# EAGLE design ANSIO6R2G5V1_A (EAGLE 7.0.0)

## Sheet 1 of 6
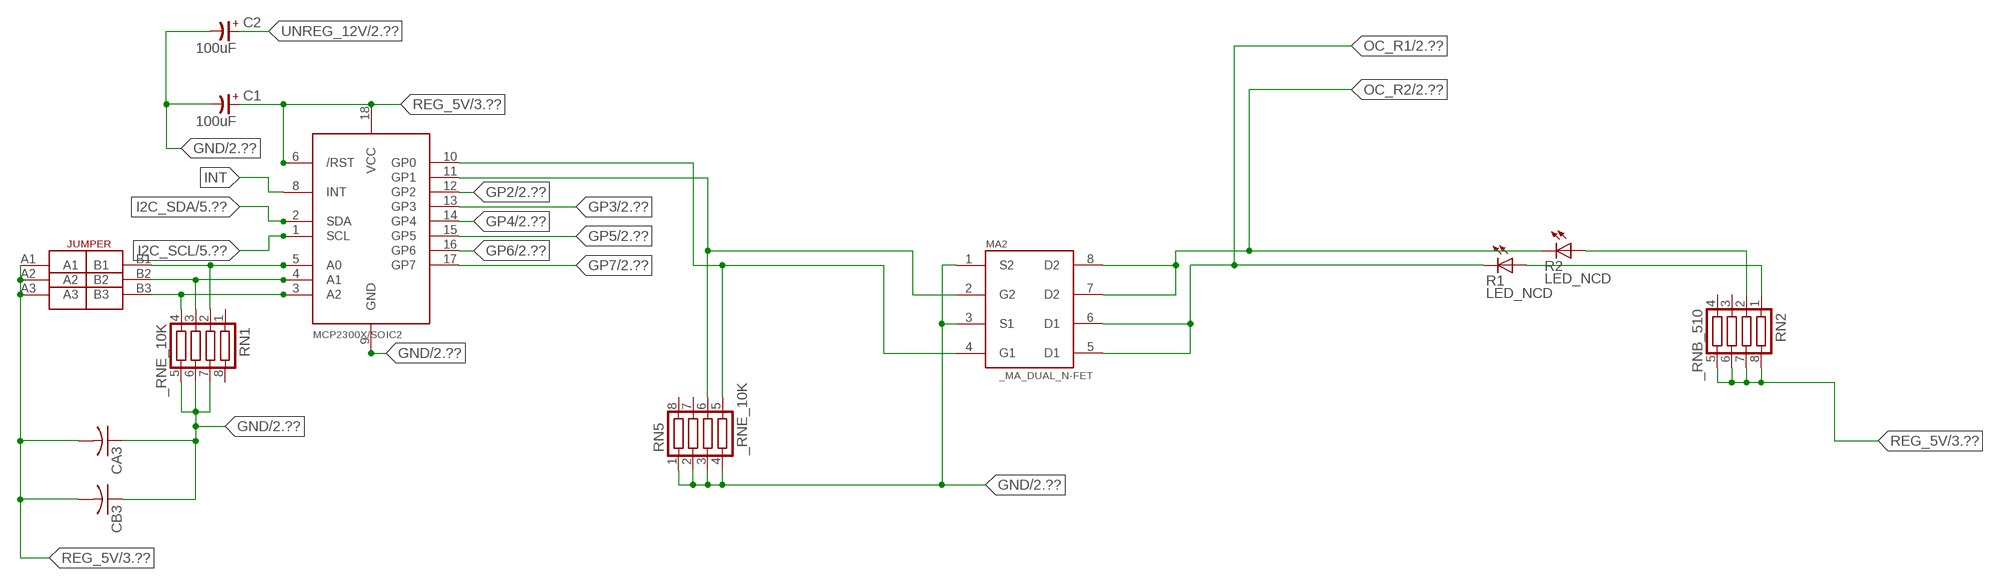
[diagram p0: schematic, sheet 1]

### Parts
C1  100uF  CP-E-025X060  [E-025X060]
C2  100uF  CP-E-025X060  [E-025X060]
CA3  CC1206KRX7R9BB104C1206K  [CC1206KRX7R9BB104]
CB3  TMK316F106ZL-TC1206K  [TMK316F106ZL-T]
IC2  MCP2300X/SO  [SO18W]
MA2  _MA_DUAL_N-FET  [_MA_DUAL_N-FET]
R1  LED_NCD  [CHIPLED_0603]
R2  LED_NCD  [CHIPLED_0603]
RN1  _RNE_10K  [RNE]
RN2  _RNB_510  [RNB]
RN5  _RNE_10K  [RNE]
U$18  JUMPER_3X2  [JUMPER_3X2]

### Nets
GND: C1.- C2.- CA3.1 CB3.1 IC2.9(GND) MA2.1(S2) MA2.3(S1) RN1.5 RN1.6 RN1.7 RN5.1 RN5.2 RN5.3 RN5.4 ; also sheet 2,3,4,5,6
GP2: IC2.12(GP2) ; also sheet 2
GP3: IC2.13(GP3) ; also sheet 2
GP4: IC2.14(GP4) ; also sheet 2
GP5: IC2.15(GP5) ; also sheet 2
GP6: IC2.16(GP6) ; also sheet 2
GP7: IC2.17(GP7) ; also sheet 2
I2C_SCL: IC2.1(SCL) ; also sheet 5,6
I2C_SDA: IC2.2(SDA) ; also sheet 5,6
INT: IC2.8(INT)
N$6: IC2.5(A0) RN1.2 U$18.B1
N$7: IC2.4(A1) RN1.3 U$18.B2
N$8: IC2.3(A2) RN1.4 U$18.B3
N$22: IC2.11(GP1) MA2.2(G2) RN5.6
N$23: IC2.10(GP0) MA2.4(G1) RN5.5
N$31: R2.A RN2.2
N$32: R1.A RN2.1
OC_R1: MA2.5(D1) MA2.6(D1) R1.C ; also sheet 2
OC_R2: MA2.7(D2) MA2.8(D2) R2.C ; also sheet 2
REG_5V: C1.+ CA3.2 CB3.2 IC2.6(/RST) IC2.18(VCC) RN2.5 RN2.6 RN2.7 RN2.8 U$18.A1 U$18.A2 U$18.A3 ; also sheet 3,4,5,6
UNREG_12V: C2.+ ; also sheet 2,3
Unconnected: RN1.1 RN1.8 RN2.3 RN2.4 RN5.7 RN5.8

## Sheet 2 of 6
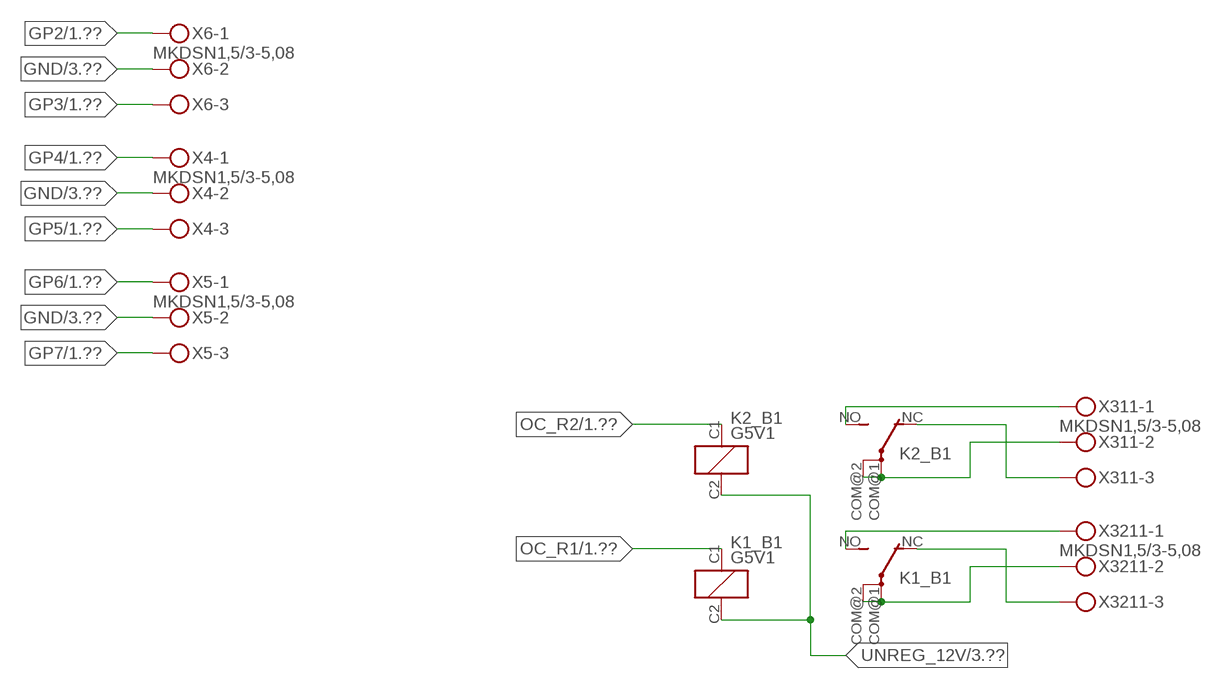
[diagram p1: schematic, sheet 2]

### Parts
K1_B1  G5V1  [G5V1]
K2_B1  G5V1  [G5V1]
X4  MKDSN1,5/3-5,08  [MKDSN1,5/3-5,08]
X5  MKDSN1,5/3-5,08  [MKDSN1,5/3-5,08]
X6  MKDSN1,5/3-5,08  [MKDSN1,5/3-5,08]
X311  MKDSN1,5/3-5,08  [MKDSN1,5/3-5,08]
X3211  MKDSN1,5/3-5,08  [MKDSN1,5/3-5,08]

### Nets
GND: X4.2 X5.2 X6.2 ; also sheet 1,3,4,5,6
GP2: X6.1 ; also sheet 1
GP3: X6.3 ; also sheet 1
GP4: X4.1 ; also sheet 1
GP5: X4.3 ; also sheet 1
GP6: X5.1 ; also sheet 1
GP7: X5.3 ; also sheet 1
N$221: K2_B1.NO(2:S) X311.1
N$222: K2_B1.NC(2:O) X311.3
N$223: K2_B1.COM@1(2:P) K2_B1.COM@2(2:P) X311.2
N$224: K1_B1.NO(2:S) X3211.1
N$225: K1_B1.NC(2:O) X3211.3
N$226: K1_B1.COM@1(2:P) K1_B1.COM@2(2:P) X3211.2
OC_R1: K1_B1.C1(1:C1) ; also sheet 1
OC_R2: K2_B1.C1(1:C1) ; also sheet 1
UNREG_12V: K1_B1.C2(1:C2) K2_B1.C2(1:C2) ; also sheet 1,3

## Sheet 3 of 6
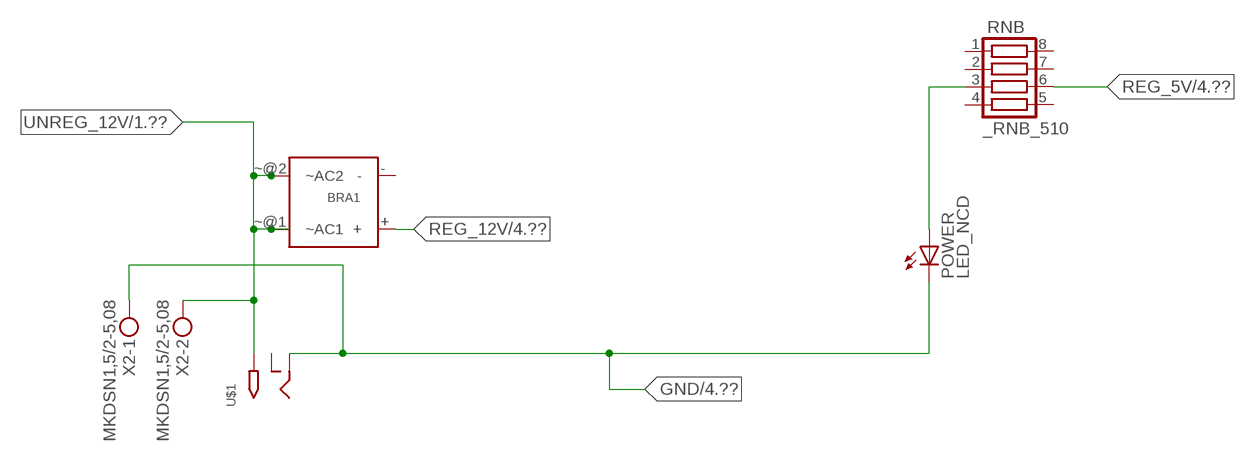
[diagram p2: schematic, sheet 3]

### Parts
BRA1  MB2S_  [MB2S]
POWER  LED_NCD  [CHIPLED_0603]
RNB  _RNB_510  [RNB]
U$1  2.1MMJACK  [PJ-102A]
X2  MKDSN1,5/2-5,08  [MKDSN1,5/2-5,08]

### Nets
GND: POWER.C U$1.RING X2.1 ; also sheet 1,2,4,5,6
N$2: POWER.A RNB.3
REG_5V: RNB.6 ; also sheet 1,4,5,6
REG_12V: BRA1.+ ; also sheet 4
UNREG_12V: BRA1.~@1(~AC1) BRA1.~@2(~AC2) U$1.TIP X2.2 ; also sheet 1,2
Unconnected: BRA1.- RNB.1 RNB.2 RNB.4 RNB.5 RNB.7 RNB.8 U$1.RING_SW

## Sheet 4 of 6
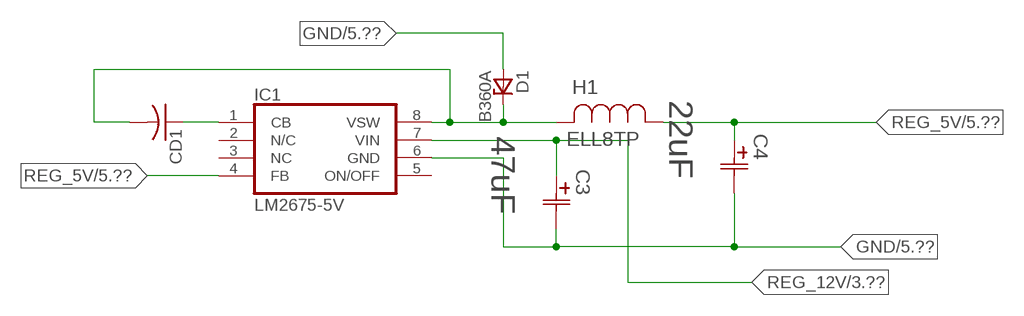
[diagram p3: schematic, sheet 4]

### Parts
C3  47uF  490-5463-6-NDCAP  [C2917(7343)-Y]
C4  22uF  490-5463-6-NDCAP  [C2917(7343)-Y]
CD1  _CD_10NF_50VC1206K  [_CD_10NF_50V]
D1  B360A  [DO214AC_ZENER]
H1  ELL8TP  [IND_ELL8TP]
IC1  LM2675-5V  LM2675  [SO-8]

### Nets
GND: C3.2(C2) C4.2(C2) D1.A IC1.6(GND) ; also sheet 1,2,3,5,6
N$1: CD1.2 D1.C H1.2 IC1.8(VSW)
N$3: CD1.1 IC1.1(CB)
REG_5V: C4.1(C1) H1.1 IC1.4(FB) ; also sheet 1,3,5,6
REG_12V: C3.1(C1) IC1.7(VIN) ; also sheet 3
Unconnected: IC1.2(N/C) IC1.5(ON/OFF)

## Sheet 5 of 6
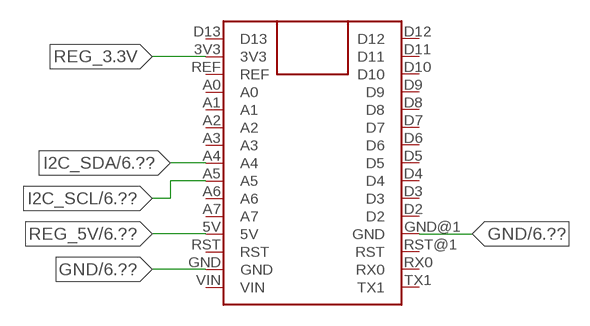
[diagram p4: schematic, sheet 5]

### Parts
FOR_NANO  ARDUINO_NANO  [ARDUINO_NANO]

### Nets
GND: FOR_NANO.GND FOR_NANO.GND@1(GND) ; also sheet 1,2,3,4,6
I2C_SCL: FOR_NANO.A5 ; also sheet 1,6
I2C_SDA: FOR_NANO.A4 ; also sheet 1,6
REG_3.3V: FOR_NANO.3V3
REG_5V: FOR_NANO.5V ; also sheet 1,3,4,6
Unconnected: FOR_NANO.A0 FOR_NANO.A1 FOR_NANO.A2 FOR_NANO.A3 FOR_NANO.A6 FOR_NANO.A7 FOR_NANO.D2 FOR_NANO.D3 FOR_NANO.D4 FOR_NANO.D5 FOR_NANO.D6 FOR_NANO.D7 FOR_NANO.D8 FOR_NANO.D9 FOR_NANO.D10 FOR_NANO.D11 FOR_NANO.D12 FOR_NANO.D13 FOR_NANO.REF FOR_NANO.RST FOR_NANO.RST@1(RST) FOR_NANO.RX0 FOR_NANO.TX1 FOR_NANO.VIN

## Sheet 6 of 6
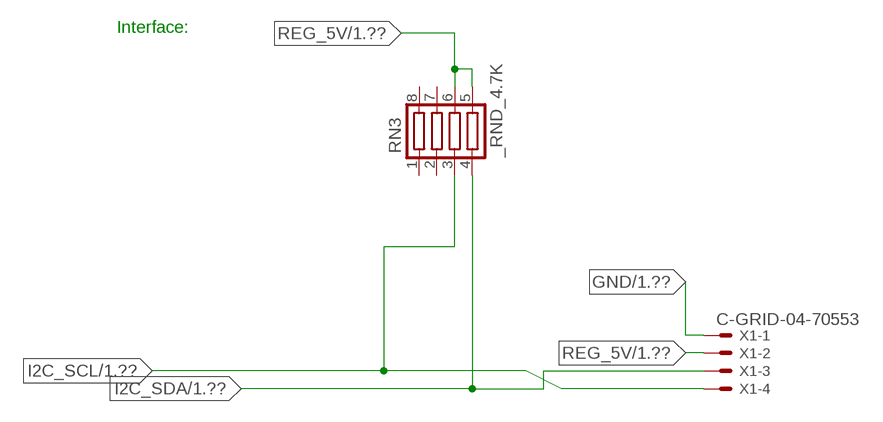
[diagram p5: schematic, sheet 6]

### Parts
RN3  _RND_4.7K  [RND]
X1  C-GRID-04-70553  [70553-04]

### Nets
GND: X1.1 ; also sheet 1,2,3,4,5
I2C_SCL: RN3.3 X1.4 ; also sheet 1,5
I2C_SDA: RN3.4 X1.3 ; also sheet 1,5
REG_5V: RN3.5 RN3.6 X1.2 ; also sheet 1,3,4,5
Unconnected: RN3.1 RN3.2 RN3.7 RN3.8

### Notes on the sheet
- Interface:

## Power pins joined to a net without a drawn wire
NC: IC1.3(NC)

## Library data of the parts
BRA1 = NCD_ULTIMATE_LIBRARY:MB2S: Bridge Rectifier BRA MB2S 200V 500ma Digikey MB2S-TPMSTR-ND/MB2S-TP
C1 C2 = NCD_ULTIMATE_LIBRARY:CP-: Capacitors All Kinds POLARIZED CAP
C3 C4 = NCD_ULTIMATE_bhaskar:490-5463-6-ND: NCD CAP
CA3 = NCD_ULTIMATE_LIBRARY:CC1206KRX7R9BB104: Capacitor CA .1uF 50V SMT C1206K CC1206KRX7R9BB104
CB3 = NCD_ULTIMATE_LIBRARY:TMK316F106ZL-T: Capacitor CB 10uF SMT 1206 TMK316F106ZL-T
CD1 = NCD_ULTIMATE_LIBRARY:_CD_10NF_50V: Capacitor 10nF SMT
D1 = NCD_ULTIMATE_bhaskar:B360A: NCD DIODE B350A/B360A
FOR_NANO = NCD_ULTIMATE_CONNECTORS:ARDUINO_NANO
H1 = NCD_ULTIMATE_bhaskar:ELL8TP: NCD coil
IC1 = NCD_ULTIMATE_bhaskar:LM2675: LM2675 NCD http://www.ti.com/lit/ds/symlink/lm2675.pdf
IC2 = NCD_ULTIMATE_LIBRARY:MCP2300X: Semiconductor Port Expander I/O 8-Bit I2C MCP23008 Inexpensive i2c i/o expander - 8 general purpose i/o pins with optional pullups
K1_B1 K2_B1 = NCD_ULTIMATE_LIBRARY:G5V1: RELAY 1 x switch, 0.5 A/125 V AC, 1 A/24 V DC , Omron
MA2 = NCD_ULTIMATE_LIBRARY:_MA_DUAL_N-FET: FET Dual N-Channel 8-SOIC NMOSFET Digikey 785-1064-2-ND/AO4842
POWER = NCD_ULTIMATE_bhaskar:LED_NCD
R1 R2 = NCD_ULTIMATE_LIBRARY:LED_NCD: LED Digikey 754-1132-2-ND/APT2012SRCPRV
RN1 RN5 = NCD_ULTIMATE_LIBRARY:_RNE_10K: Resistor Array RNE SMT 10K x 4 Single Resistor Source: http://www.ctscorp.com/components/Datasheets/CTSChipArrayDs.pdf Digikey 742C083103JPTR-ND/742C083103JP; OC_FARNELL: unknown; OC_NEWARK: unknown
RN2 RNB = NCD_ULTIMATE_LIBRARY:_RNB_510: Resistor Array RNB SMT 510 x 4 Single Resistor Source: http://www.ctscorp.com/components/Datasheets/CTSChipArrayDs.pdf Digikey 742C083511JPTR-ND/ 742C083511JP; OC_FARNELL: unknown; OC_NEWARK: unknown
RN3 = NCD_ULTIMATE_LIBRARY:_RND_4.7K: Resistor Array RND SMT 4.7K x 4 Single Resistor Source: http://www.ctscorp.com/components/Datasheets/CTSChipArrayDs.pdf Digikey 742C083472JPTR-ND/742C083472JP; OC_FARNELL: unknown; OC_NEWARK: unknown
U$1 = NCD_ULTIMATE_CONNECTORS:2.1MMJACK: 2.1mm x 5.5mm DC jack with internal switch. Digikey part #PJ-102A, 4UCON part #05537 By microbuilder.eu
U$18 = NCD_ULTIMATE_CONNECTORS:JUMPER_3X2
X1 = NCD_ULTIMATE_CONNECTORS:C-GRID-04: CONNECTOR 4-Pos I2C wire to board 2.54 mm (0.100") pitch header Digikey WM1342-ND/0015912045; OC_FARNELL: unknown; OC_NEWARK: unknown
X2 = NCD_ULTIMATE_CONNECTORS:MKDSN1,5/2-5,08: MKDSN 1,5/ 2-5,08 Printklemme
X4-X6 X311 X3211 = NCD_ULTIMATE_CONNECTORS:MKDSN1,5/3-5,08: MKDSN 1,5/ 3-5,08 Printklemme Nennstrom: 13,5 A Nennspannung: 250 V Rastermaß: 5,08 mm Polzahl: 3 Anschlussart: Schraubanschluss Montage: Löten Anschlussrichtung Leiter/Platine: 0 ° Artikelnummer: 1729131 Source: http://eshop.phoenixcontact.com .. 1729131.pdf

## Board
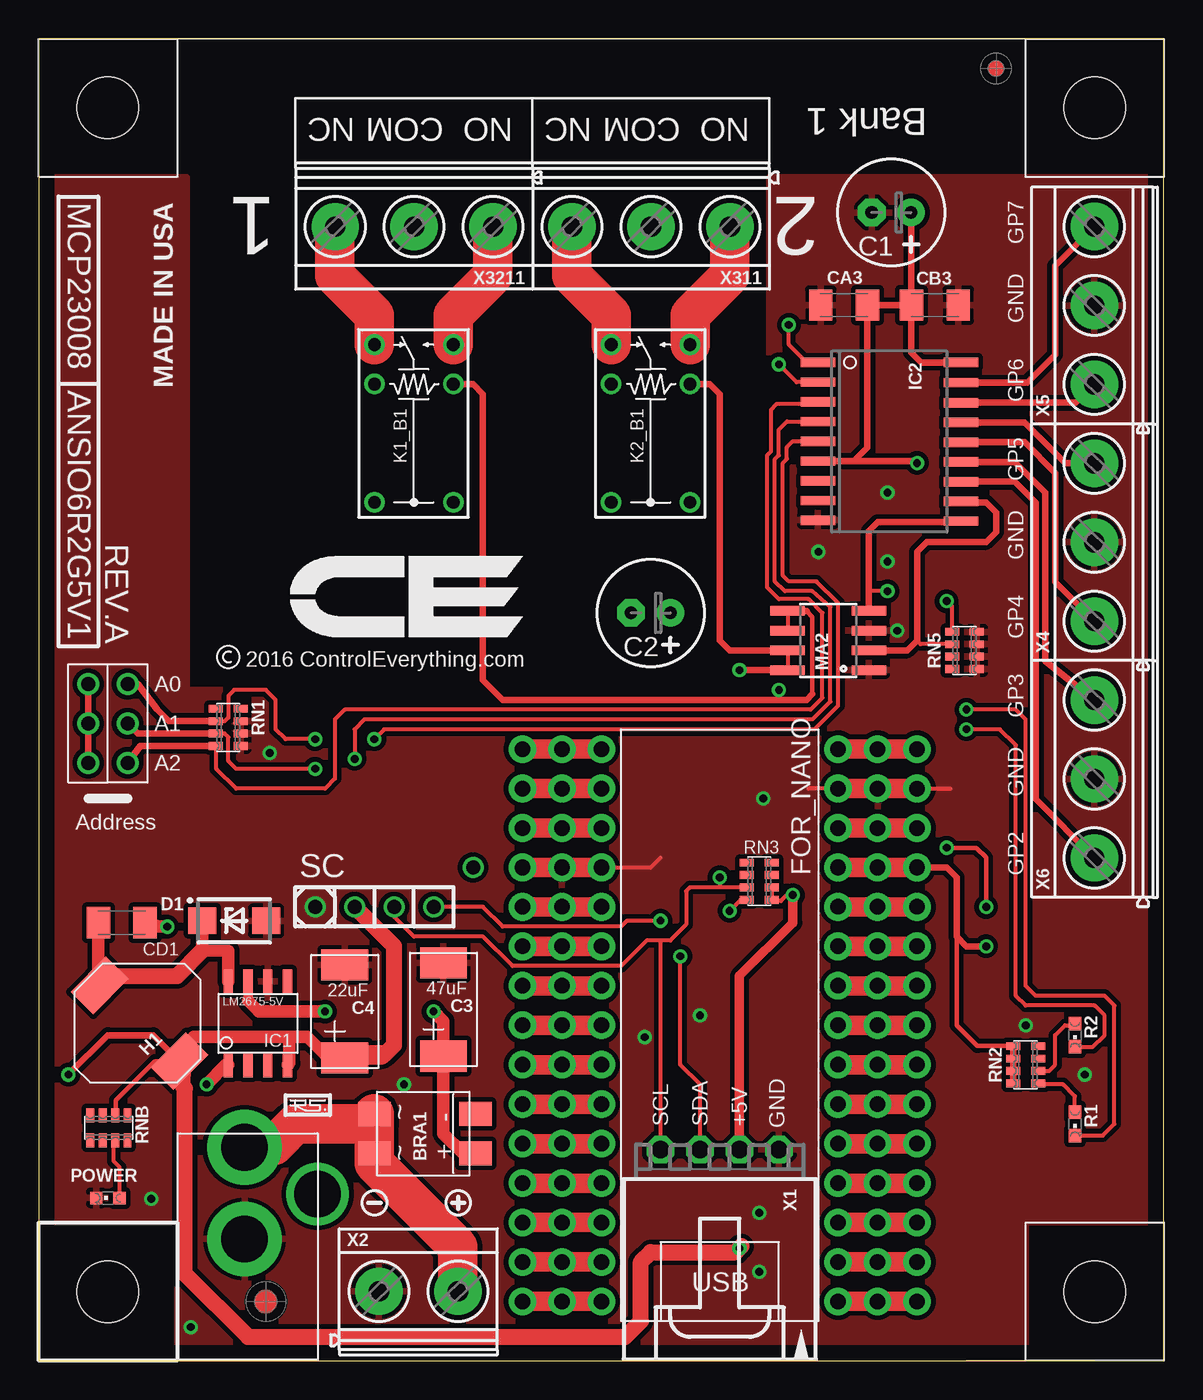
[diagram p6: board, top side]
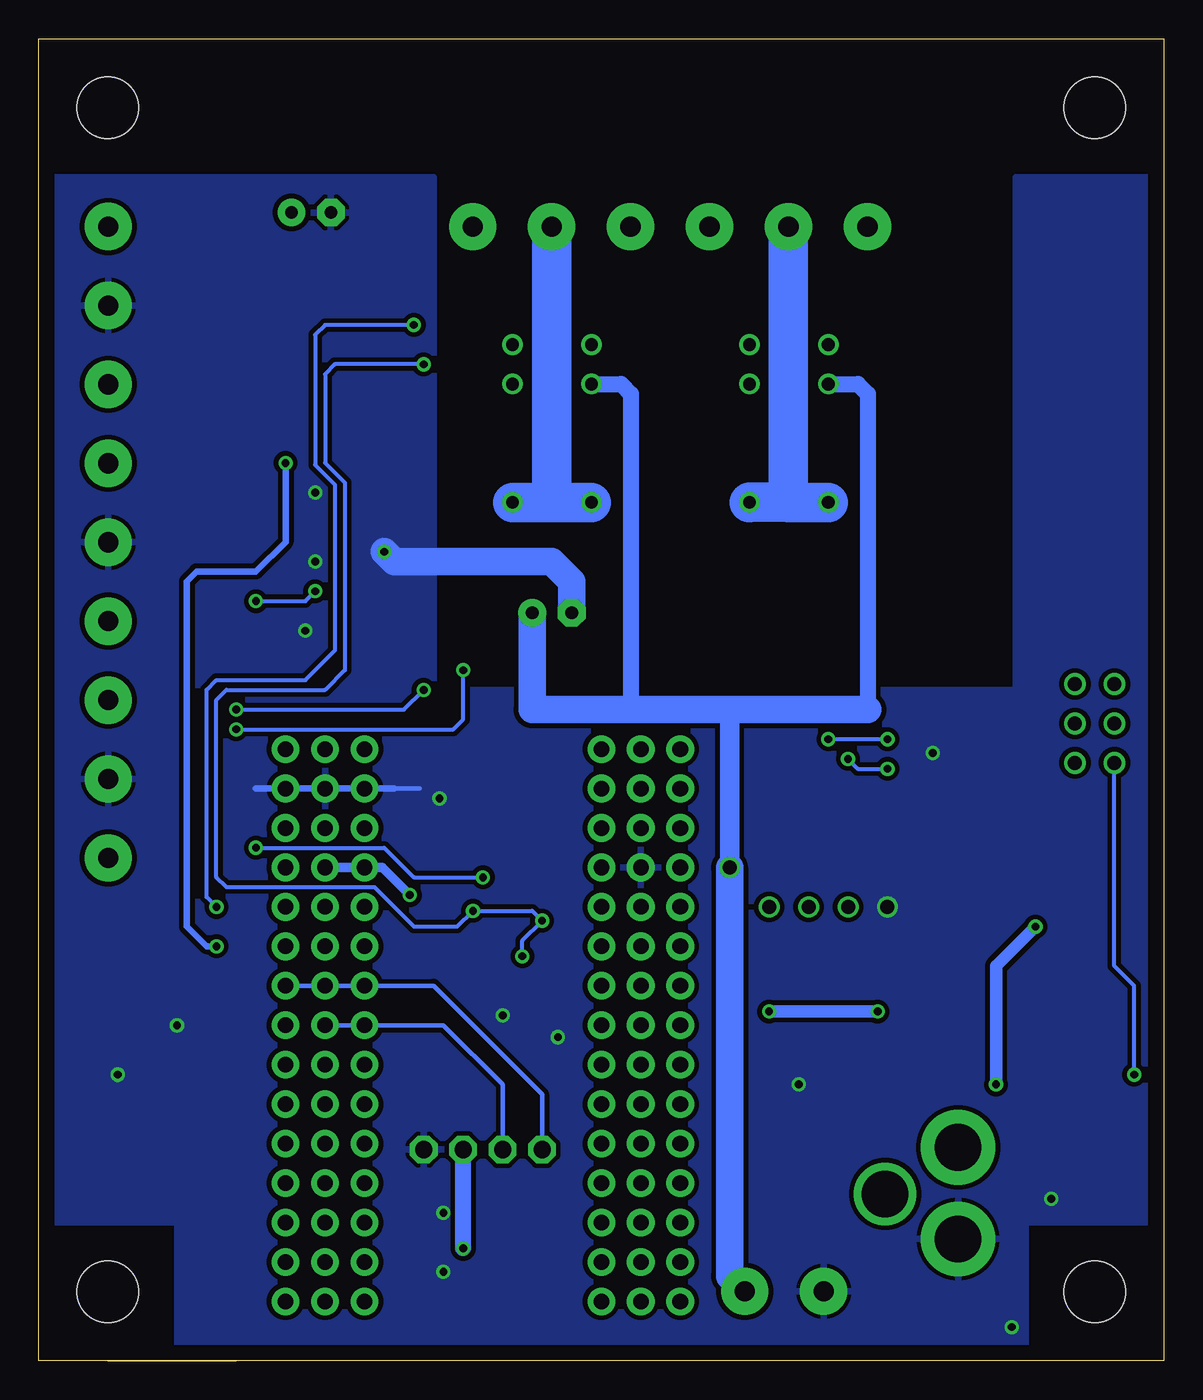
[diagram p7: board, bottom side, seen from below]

Size 72.39 x 85.09 mm. Coordinates in mm from the lower left corner, seen from the top.
Outline: 0,65.71 0,64.77
Outline: 0,64.77 0,0 59.69,0
Outline: 59.69,0 72.39,0 72.39,85.09 0,85.09 0,64.77
Outline: 67.94,0 59.69,0
Copper layers (1*16): Top 0.035mm / dielectric 1.5mm / Bottom 0.035mm
Design rules "default": minimum track width 10mil, minimum drill 24mil, track to track 8mil, track to pad 8mil, pad to pad 8mil, via to via 8mil, smd to smd 8mil, copper to edge 40mil, drill to drill 8mil, minimum pad ring 10mil, minimum via ring 8mil, stop-mask expansion 4mil, vias tented up to drill 0mil, thermal gap 10mil
Holes 3.96 mm at 4.45,4.45 4.45,4.45 4.45,4.45 4.45,4.45

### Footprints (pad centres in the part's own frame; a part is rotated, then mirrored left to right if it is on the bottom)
MB2S = smd 1.55 x 2.1: + 0,-6.5; - 2.54,-6.5; ~@1 0,0; ~@2 2.54,0
E-025X060 = drill 0.813 pad 1.778: + -1.27,0 | drill 0.813 pad 1.778 octagon: - 1.27,0
C2917(7343)-Y = smd 2 x 3: 1 -3,0; 2 3,0
CC1206KRX7R9BB104 = smd 1.5 x 2: 1 -1.5,0; 2 1.5,0
TMK316F106ZL-T = smd 1.5 x 2: 1 -1.5,0; 2 1.5,0
_CD_10NF_50V = smd 1.5 x 2: 1 -1.5,0; 2 1.5,0
DO214AC_ZENER = smd 1.8 x 1.7: A 2.05,0; C -2.05,0
ARDUINO_NANO = drill 1 pad 1.778: 3V1 -2.54,-2.54; 3V3 0,-2.54; 5V 0,-27.94; 5V1 -2.54,-27.94; A0 0,-7.62; A1 0,-10.16; A2 0,-12.7; A3 0,-15.24; A4 0,-17.78; A5 0,-20.32; A6 0,-22.86; A7 0,-25.4; A8 -2.54,-7.62; A9 -2.54,-10.16; A10 -2.54,-12.7; A11 -2.54,-15.24; A12 -2.54,-17.78; A13 -2.54,-20.32; A14 -2.54,-22.86; A15 -2.54,-25.4; D1 -2.54,0; D2 20.32,-25.4; D3 20.32,-22.86; D4 20.32,-20.32; D5 20.32,-17.78; D6 20.32,-15.24; D7 20.32,-12.7; D8 20.32,-10.16; D9 20.32,-7.62; D10 20.32,-5.08; D11 20.32,-2.54; D12 20.32,0; D13 0,0; D14 22.86,0; D15 22.86,-2.54; D16 22.86,-5.08; D17 22.86,-7.62; D18 22.86,-10.16; D19 22.86,-12.7; D20 22.86,-15.24; D21 22.86,-17.78; D22 22.86,-20.32; D23 22.86,-22.86; D24 22.86,-25.4; GND 0,-33.02; GND1 -2.54,-33.02; GND@1 20.32,-27.94; GND@2 22.86,-27.94; P$16 2.54,0; P$17 2.54,-2.54; P$18 2.54,-5.08; P$19 2.54,-7.62; P$20 2.54,-10.16; P$21 2.54,-12.7; P$22 2.54,-15.24; P$23 2.54,-17.78; P$24 2.54,-20.32; P$25 2.54,-22.86; P$26 2.54,-25.4; P$27 2.54,-27.94; P$28 2.54,-30.48; P$29 2.54,-33.02; P$30 2.54,-35.56; P$31 17.78,0; P$32 17.78,-2.54; P$33 17.78,-5.08; P$34 17.78,-7.62; P$35 17.78,-10.16; P$36 17.78,-12.7; P$37 17.78,-15.24; P$38 17.78,-17.78; P$39 17.78,-20.32; P$40 17.78,-22.86; P$41 17.78,-25.4; P$42 17.78,-27.94; P$43 17.78,-30.48; P$44 17.78,-33.02; P$45 17.78,-35.56; REF 0,-5.08; REF1 -2.54,-5.08; RST 0,-30.48; RST1 -2.54,-30.48; RST@1 20.32,-30.48; RST@2 22.86,-30.48; RX0 20.32,-33.02; RX1 22.86,-33.02; TX1 20.32,-35.56; TX2 22.86,-35.56; VIN 0,-35.56; VIN1 -2.54,-35.56
IND_ELL8TP = smd 2.054 x 3.2 rotated 45: 1 -2.442,-2.696; 2 2.442,2.442
SO-8 = smd 0.6 x 1.55: 1 -1.905,-2.69; 2 -0.635,-2.69; 3 0.635,-2.69; 4 1.905,-2.69; 5 1.905,2.71; 6 0.635,2.71; 7 -0.635,2.71; 8 -1.905,2.71
SO18W = smd 0.6 x 2.2: 1 -4.445,-4.6; 2 -3.175,-4.6; 3 -1.905,-4.6; 4 -0.635,-4.6; 5 0.635,-4.6; 6 1.905,-4.6; 7 3.175,-4.6; 8 4.445,-4.6; 9 5.715,-4.6; 10 5.775,4.6; 11 4.505,4.6; 12 3.235,4.6; 13 1.965,4.6; 14 0.695,4.6; 15 -0.575,4.6; 16 -1.845,4.6; 17 -3.145,4.6; 18 -4.445,4.6
G5V1 = drill 0.813: C1 -2.54,2.54; C2 -2.54,-2.54; COM@1 5.08,-2.54; COM@2 5.08,2.54; NC -5.08,-2.54; NO -5.08,2.54
_MA_DUAL_N-FET = smd 0.61 x 2.21: 1 -1.905,-2.616; 2 -0.635,-2.616; 3 0.635,-2.616; 4 1.905,-2.616; 5 1.905,2.616; 6 0.635,2.616; 7 -0.635,2.616; 8 -1.905,2.616
CHIPLED_0603 = smd 0.8 x 0.8: A 0,-0.75; C 0,0.75
CHIPLED_0603' = smd 0.8 x 0.876: A 0,-0.75; C 0,0.75
RNE = smd 0.5 x 0.9: 1 -1.2,-0.8; 2 -0.4,-0.8; 3 0.4,-0.8; 4 1.2,-0.8; 5 1.2,0.8; 6 0.4,0.8; 7 -0.4,0.8; 8 -1.2,0.8
RNB = smd 0.5 x 0.9: 1 -1.2,-0.8; 2 -0.4,-0.8; 3 0.4,-0.8; 4 1.2,-0.8; 5 1.2,0.8; 6 0.4,0.8; 7 -0.4,0.8; 8 -1.2,0.8
RND = smd 0.5 x 0.9: 1 -1.2,-0.8; 2 -0.4,-0.8; 3 0.4,-0.8; 4 1.2,-0.8; 5 1.2,0.8; 6 0.4,0.8; 7 -0.4,0.8; 8 -1.2,0.8
PJ-102A = drill 3 pad 4.8: RING 0.1,-3.39; TIP 0.1,-9.29 | drill 3 pad 3.251: RING_SW -4.6,-6.29
PCB_MOUNTING_HOLE = hole 3.962: 4.445,4.445
JUMPER_3X2 = drill 0.9: A1 0,5.08; A2 0,2.54; A3 0,0; B1 2.54,5.08; B2 2.54,2.54; B3 2.54,0
70553-04 = drill 1.1 pad 1.778 octagon: 1 -3.81,-7.62; 2 -1.27,-7.62; 3 1.27,-7.62; 4 3.81,-7.62
MKDSN1,5/2-5,08 = drill 1.3 pad 3.048: 1 -2.561,0.025; 2 2.519,0.025
MKDSN1,5/3-5,08 = drill 1.3 pad 3.048: 1 -7.641,0.025; 2 -2.561,0.025; 3 2.519,0.025

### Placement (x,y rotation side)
BRA1  21.59,13.34 90 top
C1  54.86,73.91 180 top
C2  39.37,48.13 180 top
C3  26.04,22.61 90 top
C4  19.68,22.48 90 top
CA3  51.82,67.94 0 top
CB3  57.66,67.94 180 top
CD1  5.33,28.19 180 top
D1  12.57,28.32 0 top
FOR_NANO  53.98,3.81 180 top
H1  6.35,21.72 90 top
IC1  14.1,21.72 0 top
IC2  54.74,59.82 270 top
K1_B1  24.13,60.33 270 top
K2_B1  39.37,60.33 270 top
MA2  50.8,46.36 90 top
POWER  4.45,10.48 90 top
R1  LED_NCD  [CHIPLED_0603']  66.67,15.24 180 top
R2  LED_NCD  [CHIPLED_0603']  66.67,20.95 180 top
RN1  12.19,40.77 270 top
RN2  63.5,19.05 90 top
RN3  46.35,30.86 270 top
RN5  59.56,45.72 90 top
RNB  4.51,14.99 0 top
U$1  13.34,4.45 180 top
U$2  [VISION_REF15]  14.61,3.81 0 top
U$3  [ICON_MINUS]  21.59,10.16 180 top
U$4  PCB_MOUNTING_HOLE  [PCB_MOUNTING_HOLE]  72.39,76.2 90 top
U$5  [ICON_PLUS]  26.99,10.16 90 top
U$6  PCB_MOUNTING_HOLE  [PCB_MOUNTING_HOLE]  72.39,0 90 top
U$11  PCB_MOUNTING_HOLE  [PCB_MOUNTING_HOLE]  8.89,76.2 90 top
U$18  3.17,38.48 0 top
U$19  [VISION_REF10]  61.59,83.19 0 top
U$21  [ICON_USA]  7.37,74.55 270 top
X1  43.81,5.97 180 top
X2  24.45,4.45 0 top
X4  67.94,55.24 90 top
X5  67.94,70.48 90 top
X6  67.94,40 90 top
X311  36.83,73.03 180 top
X3211  21.59,73.03 180 top

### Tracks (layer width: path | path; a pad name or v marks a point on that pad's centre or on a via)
GND  (via drill 0.5, 0.9)
  Top 0.254: 36.2,31.75 39.37,31.75 40.01,32.39 | FOR_NANO.GND@1 32.38,31.75 | 49.53,36.83 56.52,36.83 58.67,36.83
  Top 1.016: X1.1 47.62,13.74
  Bottom 0.254: 51.44,36.83 FOR_NANO.GND
  Bottom 0.305: 47.88,36.83 49.53,36.83 51.44,36.83
  Bottom 0.406: 49.53,36.83 58.42,36.83
  Bottom 1.778: C2.- 38.1,50.16 39.37,51.44 49.53,51.44 v50.16,52.07
  other vias: 14.86,39.12 54.61,51.44 54.61,55.88 63.5,21.59 67.31,18.41 55.24,46.99 9.78,2.16 17.78,29.21 46.35,9.53 46.61,36.2 46.35,5.72 42.55,22.23 38.99,20.83 7.24,10.41 23.5,17.78
  pour Bottom (isolate 0.305): -3.81,8.89 8.89,8.89 8.89,0 63.5,0 63.5,8.89 71.75,8.89 71.75,76.2 46.99,76.2 46.99,43.18 9.53,43.18 9.53,76.2 -3.81,76.2
  pour Top (isolate 0.305): -8.26,8.89 8.89,8.89 8.89,0 63.5,0 63.5,8.89 71.75,8.89 71.75,76.2 46.99,76.2 46.99,43.18 9.53,43.18 9.53,76.2 -8.26,76.2
GP2
  Top 0.406: IC2.12 62.8,56.58 64.14,55.24 64.14,36.15 X6.1
GP3
  Top 0.406: IC2.13 62.8,57.85 64.77,55.88 64.77,45.04 X6.3
GP4
  Top 0.406: IC2.14 63.43,59.12 65.41,57.15 65.41,50.12 X4.1
GP5
  Top 0.406: IC2.15 63.43,60.39 66.04,57.79 67.9,57.79 X4.3
GP6
  Top 0.406: IC2.16 66.74,61.66 X5.1
GP7
  Top 0.406: IC2.17 63.6,62.96 65.41,64.77 65.41,70.49 X5.3
I2C_SCL  (via drill 0.5, 0.9)
  Top 0.254: IC2.1 49.4,64.26 48.26,65.41 v48.26,66.67 | 40.01,27.05 40.64,27.05 41.66,28.07 41.66,30.23 41.89,30.46 RN3.3 45.54,30.48 43.81,30.48 v43.81,31.12 | 40.01,27.05 39.12,27.05 37.47,25.4 30.48,25.4 28.57,27.3 24.13,27.3 22.86,28.57 v22.86,29.21 | X1.4 40.01,27.05
  Top 0.305: v60.96,29.21 60.96,32.39 60.33,33.02 v58.42,33.02
  Bottom 0.254: v48.26,66.67 53.98,66.67 54.61,66.04 54.61,57.66 53.34,56.39 53.34,45.72 55.24,43.81 60.96,43.81 61.59,43.18 61.59,29.84 v60.96,29.21 | v58.42,33.02 50.16,33.02 48.26,31.12 v43.81,31.12 | 51.44,24.13 FOR_NANO.A5
  Bottom 0.305: X1.4 40.01,17.15 46.99,24.13 FOR_NANO.A5 56.52,24.13
I2C_SDA  (via drill 0.5, 0.9)
  Top 0.254: IC2.2 48.77,62.99 v47.62,64.13 | RN3.4 45.16,29.66 v44.45,28.96 | 40,28.33 v40.01,28.32 37.85,28.32 37.47,27.94 29.84,27.94 28.57,29.21 v25.4,29.21 | X1.3 42.55,17.78 41.27,19.05 v41.27,26.04
  Bottom 0.254: v47.62,64.13 53.34,64.13 53.98,63.5 53.98,57.79 52.7,56.52 52.7,44.45 53.98,43.18 60.33,43.18 60.96,42.55 60.96,31.12 60.33,30.48 50.8,30.48 48.26,27.94 45.47,27.94 v44.45,28.96 40.64,28.96 v40.01,28.32 41.27,27.05 v41.27,26.04
  Bottom 0.305: FOR_NANO.A4 46.35,21.59 42.55,17.78 X1.3
N$1
  Top 0.813: H1.2 3.88,24.77 | D1.C 10.52,26.4 12.19,26.38 IC1.8 | CD1.2 3.83,24.15 4.45,24.77
  Top 1.016: 3.88,24.77 4.45,24.77 8.89,24.77 10.52,26.4
N$2
  Top 0.254: POWER.A 5.2,12.46 4.83,12.83 4.83,14.1 RNB.3
  Top 0.406: 4.95,14.14 RNB.3
N$3  (via drill 0.5)
  Top 0.813: IC1.1 12.04,19.03 v10.79,17.78 | v8.26,27.94 7.72,27.94 CD1.1
  Bottom 0.813: v10.79,17.78 10.79,25.4 v8.26,27.94
N$6  (via drill 0.5)
  Top 0.254: v21.59,40 22.23,40.64 49.91,40.64 51.44,42.16 51.44,48.77 50.04,50.16 48.26,50.16 47.88,50.55 47.88,57.79 48.13,58.04 48.13,58.8 48.51,59.18 IC2.5 50.01,59.05 | v17.78,40 15.88,40 15.24,40.64 15.24,42.55 14.61,43.18 12.57,43.18 12.19,42.8 12.19,41.4 11.94,41.15 11.41,41.15 RN1.2
  Top 0.406: RN1.2 8.36,41.17 7.62,41.91 6.35,43.56 U$18.B1
  Bottom 0.254: v21.59,40 v17.78,40
N$7  (via drill 0.5)
  Top 0.254: v20.32,38.73 20.32,40.64 20.95,41.27 49.78,41.27 50.93,42.42 50.93,48.51 49.78,49.53 48.01,49.53 47.37,50.16 47.37,58.04 47.62,58.29 47.62,59.94 48.13,60.45 IC2.4 50.01,60.33 | v17.78,38.1 12.7,38.1 12.19,38.61 12.19,40.13 11.94,40.39 11.41,40.39 RN1.3
  Top 0.406: RN1.3 6.37,40.37 U$18.B2
  Bottom 0.254: v20.32,38.73 19.68,38.1 v17.78,38.1
N$8
  Top 0.254: RN1.4 11.43,39.53 11.43,38.1 12.7,36.83 18.41,36.83 19.05,37.47 19.05,41.27 19.68,41.91 49.66,41.91 50.42,42.67 50.42,48.13 49.53,49.02 47.62,49.02 46.86,49.78 46.86,58.29 47.12,58.55 47.12,61.21 47.5,61.59 50.01,61.59 IC2.3
  Top 0.406: RN1.4 6.53,39.57 U$18.B3
N$22
  Top 0.254: RN5.6 56.75,46.12 56.52,46.36
  Top 0.406: MA2.2 55.88,45.72 56.52,46.36 56.52,52.07 57.15,52.7 60.96,52.7 61.59,53.34 61.59,54.61 60.96,55.24 59.4,55.24 IC2.11
N$23  (via drill 0.5)
  Top 0.254: RN5.5 58.76,48.55 v58.42,48.9 | v54.61,49.53 53.42,49.53
  Top 0.406: MA2.4 53.42,49.53 53.42,53.42 53.98,53.98 59.27,53.98 IC2.10
  Bottom 0.254: v58.42,48.9 55.24,48.9 v54.61,49.53
N$31
  Top 0.254: RN2.2 65,18.65 65.41,19.05 65.41,20.95 66.04,21.59 66.56,21.59 R2.A
N$32
  Top 0.254: R1.A 66.67,17.02 65.91,17.78 64.37,17.78 RN2.1
N$221
  Top 2.54: K2_B1.NO 41.91,67.31 44.45,69.85 44.45,72.98 X311.1
N$222
  Top 2.54: K2_B1.NC 36.83,67.31 34.29,69.85 34.29,72.98 X311.3
N$223
  Bottom 2.54: K2_B1.COM@1 39.37,55.24 | K2_B1.COM@2 39.37,55.24 | 39.37,55.24 39.37,72.98 X311.2
N$224
  Top 2.54: K1_B1.NO 26.67,67.31 29.21,69.85 29.21,72.98 X3211.1
N$225
  Top 2.54: K1_B1.NC 21.59,67.31 19.05,69.85 19.05,72.98 X3211.3
N$226
  Bottom 2.54: X3211.2 24.15,55.27 | 24.15,55.27 24.13,55.24 K1_B1.COM@1 | 24.15,55.27 26.65,55.27 K1_B1.COM@2
OC_R1  (via drill 0.5)
  Top 0.254: MA2.5 MA2.6 | R1.C 68.47,14.49 69.22,15.24 69.22,22.86 68.58,23.5 64.14,23.5 63.5,24.13 63.5,41.27 62.87,41.91 v59.69,41.91 | v47.62,43.18 47.62,42.55
  Top 0.305: 49.4,48.26 49.78,47.88 49.78,42.93
  Top 0.406: MA2.5 49.4,48.26 | 49.78,42.93 49.4,42.55 47.62,42.55 29.84,42.55 28.57,43.81 28.57,62.23 27.94,62.87 K1_B1.C1
  Bottom 0.254: v59.69,41.91 48.9,41.91 v47.62,43.18
OC_R2  (via drill 0.5)
  Top 0.254: MA2.7 MA2.8 | R2.C 67.83,20.2 68.58,20.95 68.58,22.23 67.94,22.86 63.5,22.86 62.87,23.5 62.87,39.62 61.85,40.64 v59.69,40.64
  Top 0.406: K2_B1.C1 43.18,62.87 43.81,62.23 43.81,46.36 44.45,45.72 MA2.7 | MA2.8 v45.09,44.45
  Bottom 0.254: v59.69,40.64 45.72,40.64 45.09,41.27 v45.09,44.45
REG_5V  (via drill 0.5, 0.9)
  Top 0.254: RN3.6 RN3.5 47.23,29.59 47.75,29.59 48.13,29.97 v48.51,29.97
  Top 0.305: H1.1 7.46,19.27 4.95,16.76 4.95,15.83 RNB.6 | RN2.5 60.4,20.25 59.05,21.59 59.05,27.3
  Top 0.406: U$18.A3 U$18.A2 U$18.A1 | RN2.8 RN2.7 RN2.6 RN2.5 | IC2.18 56.77,64.26 56.13,64.9 56.13,67.92 | 56.13,67.92 CB3.2 CA3.2 53.32,58.78 52.45,57.91 IC2.6 56.39,57.91 v56.52,57.79 | C1.+ 56.13,67.92 | v1.91,18.41 4.45,20.95 7.37,20.95 H1.1 | v60.96,26.67 59.69,26.67 59.05,27.3 59.05,31.12 58.42,31.75 56.52,31.75
  Top 0.61: FOR_NANO.5V 56.52,31.75 | v48.51,29.97 48.51,28.19 45.09,24.77 X1.2
  Top 0.813: 16.13,20.83 9.96,20.83 H1.1 | 16.13,20.83 17.27,20.83 18.41,19.69 20.75,19.69 C4.1 | IC1.4 16.13,19.15 16.13,20.83
  Top 1.016: H1.1 9.27,18.41 9.27,17.65 9.4,17.53 9.4,5.59 13.46,1.52 37.72,1.52 38.73,2.54 38.73,6.35 39.37,6.99 44.83,6.99 v45.09,7.24 45.21,7.37 | 22.05,19.69 22.23,19.69 22.86,20.32 22.86,26.67 v20.32,29.21
  Top 1.27: 20.75,19.69 22.05,19.69
  Bottom 0.254: U$18.A3 3.17,25.4 1.91,24.13 v1.91,18.41
  Bottom 0.406: v56.52,57.79 56.52,52.7 58.42,50.8 62.23,50.8 62.87,50.16 62.87,27.94 61.59,26.67 v60.96,26.67
  Bottom 0.61: FOR_NANO.5V 50.29,31.75 v48.51,29.97
  Bottom 1.016: v45.09,7.24 X1.2
REG_12V  (via drill 0.5)
  Top 0.61: IC1.7 13.46,23.16 | 14.1,22.48 14.15,22.48
  Top 0.813: v18.41,22.48 14.15,22.48 13.46,23.16 | v25.4,22.48 26.04,21.84 C3.1 26.04,14.61 27.3,13.34 BRA1.+
  Bottom 0.813: v18.41,22.48 v25.4,22.48
UNREG_12V  (via drill 0.9)
  Top 2.54: X2.2 26.97,7.32 21.59,12.7 BRA1.~@1 21.59,15.24 | 21.59,15.24 BRA1.~@2 | U$1.TIP 15.14,13.87 16.51,15.24 21.59,15.24
  Bottom 1.016: K1_B1.C2 19.68,62.87 19.05,62.23 19.05,41.91 | K2_B1.C2 34.92,62.87 34.29,62.23 34.29,42.55 33.66,41.91
  Bottom 1.27: v27.94,31.75 27.94,41.91
  Bottom 1.778: 19.05,41.91 27.94,41.91 33.66,41.91 40.64,41.91 C2.+ | v27.94,31.75 27.94,5.44 X2.2

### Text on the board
tNames: Bank 1 | NC | COM | NO | NC | COM | NO | MCP23008 | 1 | 2 | GP7 | GND | ANSIO6R2G5V1 | GP6 | GP5 | REV.A | GND | GP4 | 2016 ControlEverything.com | A0 | GP3 | A1 | A2 | GND | Address | SC | GP2 | SCL | SDA | +5V | GND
